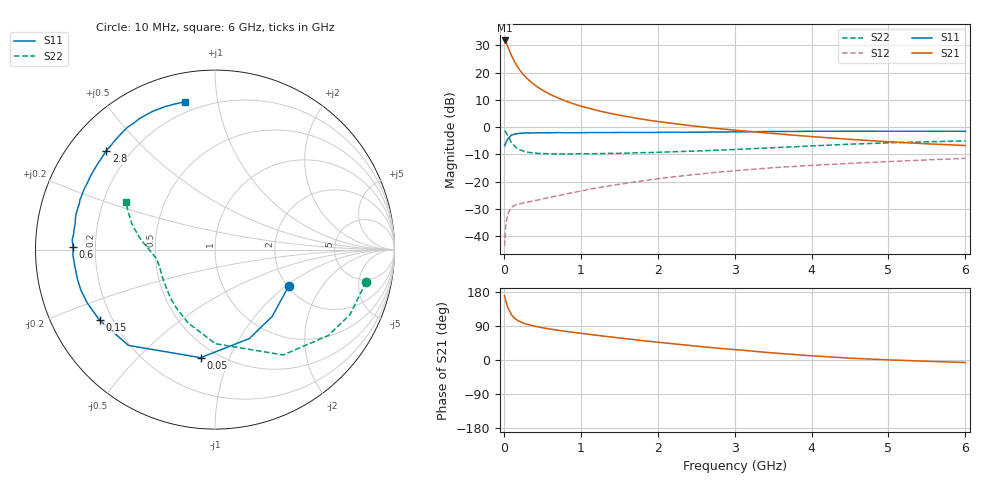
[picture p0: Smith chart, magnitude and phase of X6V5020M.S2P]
! SIEMENS Small Signal Semiconductors
! BFP193W
! Si NPN RF Bipolar Junction Transistor in SOT343
! VCE = 0.5 V  IC = 20 mA
! Common Emitter S-Parameters:  April 1994
# GHz  S  MA  R  50
!  f  S11  S21  S12  S22
! GHz  MAG  ANG  MAG  ANG  MAG  ANG  MAG  ANG
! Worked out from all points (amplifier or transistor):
!   40 points, 10 MHz to 6 GHz, reference 50 ohm
!   highest |S21| = 31.8 dB at 10 MHz (marker M1)
!   |S21| within 3 dB of that: start of sweep to 62.69 MHz
!   unconditionally stable (mu >= 1): 681 MHz to end of sweep
!   at 200 MHz: K = 0.42, MSG = 24.7 dB, |S12| = -28.1 dB
!   at 1.5 GHz: K = 1.27, MAG = 9.6 dB, |S12| = -20.9 dB
!   at 6 GHz: K = 1.14, MAG = 0.1 dB, |S12| = -11.4 dB
!   S11 on the Smith chart (normalised r, x): 10 MHz: 2.04, -1.04; 50 MHz: 0.41, -0.79; 150 MHz: 0.15, -0.28; 600 MHz: 0.12, +0.01; 2.8 GHz: 0.11, +0.38; 6 GHz: 0.14, +0.81
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0.01  0.4581 -26.2  38.95 169.6  0.0066 79.7  0.8609 -12.1
0.02  0.4902 -49.5  37.49 161.1  0.0126 71.8  0.835 -25.7
0.03  0.5313 -68.9  35.61 152.9  0.0179 65.7  0.7919 -37.2
0.05  0.6074 -97.5  30.45 139.0  0.0256 53.2  0.6993 -57.1
0.1  0.7194 -132.1  20.6 119.1  0.0343 37.9  0.5246 -89.7
0.15  0.7536 -148.6  14.88 108.3  0.0377 31.9  0.4359 -109.9
0.2  0.771 -157.2  11.49 102.1  0.0393 30.1  0.391 -123.1
0.25  0.7806 -163.2  9.366 97.7  0.0409 30.3  0.367 -132.3
0.3  0.7834 -167.3  7.838 94.5  0.0421 31.1  0.3501 -139.2
0.4  0.7869 -173.4  5.948 89.2  0.045 33.1  0.3353 -148.2
0.5  0.7919 -177.7  4.791 85.2  0.0483 36.1  0.3292 -154.0
0.6  0.7907 179.1  4.004 81.7  0.0518 38.7  0.3255 -158.4
0.8  0.7925 173.6  3.028 75.7  0.0595 43.1  0.3231 -163.5
1.1  0.7975 167.2  2.237 67.9  0.0722 47.3  0.3264 -168.3
1.3  0.7984 163.2  1.903 62.9  0.0811 48.8  0.3299 -170.2
1.6  0.8015 157.6  1.568 55.8  0.0946 49.9  0.3349 -172.7
2.2  0.8069 147.4  1.172 42.8  0.1228 49.0  0.3549 -177.5
2.8  0.8189 137.7  0.941 30.9  0.1504 46.1  0.3809 178.0
3.2  0.8265 131.5  0.836 24.0  0.168 43.5  0.4022 174.4
4.5  0.8451 114.4  0.599 4.9  0.2175 34.2  0.4887 162.3
5.5  0.8416 105.7  0.497 -3.3  0.2517 27.7  0.5404 154.7
6  0.8408 101.3  0.462 -6.6  0.2689 24.8  0.562 151.6
